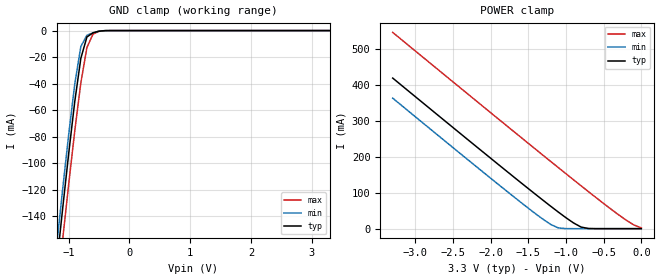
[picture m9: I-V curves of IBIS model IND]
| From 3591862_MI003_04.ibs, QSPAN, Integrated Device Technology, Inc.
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|   Model IND
[Model]   IND
Model_type   Input
Polarity   Non-Inverting
Vinl =   0.8000V
Vinh =   2.0000V
C_comp   5.0000pF   5.0000pF   5.0000pF
[Temperature Range]   27.0000   0.000   70.0000
[Voltage Range]   3.3000V   3.0000V   4.0000V
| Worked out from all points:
|   GND clamp passes 1 mA (typ) near -0.54 V on its own axis
|   POWER clamp passes 1 mA (typ) near -0.71 V on its own axis
[GND_clamp]
| voltage   I(typ)   I(min)   I(max)
-3.3V     -1.137A    -1.124A    -1.159A
-1.2V     -178mA     -163.4mA   -201.5mA
-1.1V     -134.8mA   -120.2mA   -158.2mA
-1V       -92.89mA   -78.57mA   -116.1mA
-900mV    -53.62mA   -40.34mA   -75.79mA
-800mV    -20.94mA   -12.05mA   -39.44mA
-700mV    -4.835mA   -3.507mA   -12.8mA
-600mV    -1.724mA   -1.656mA   -2.668mA
-500mV    -436.7uA   -367.2uA   -590.4uA
-400mV    -40.4uA    -22.34uA   -82.64uA
3.3V      120.9pA    105.8pA    309.4pA
[POWER_clamp]
| voltage   I(typ)   I(min)   I(max)
-3.3V     417.9mA    362.2mA    544.7mA
-1.7V     144.7mA    89.68mA    270.8mA
-1.4V     94.56mA    40.8mA     219.8mA
-1.2V     61.77mA    11.38mA    186mA
-1.1V     45.78mA    1.897mA    169.2mA
-900mV    15.9mA     9.943uA    135.6mA
-800mV    4.474mA    383nA      119mA
-700mV    390.7uA    10.32nA    102.4mA
-200mV    242.9pA    103.4pA    23.45mA
-100mV    127.6pA    101pA      10.4mA
0V        120.9pA    98.55pA    2.021mA
